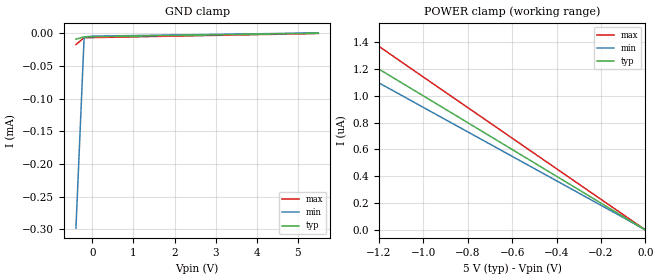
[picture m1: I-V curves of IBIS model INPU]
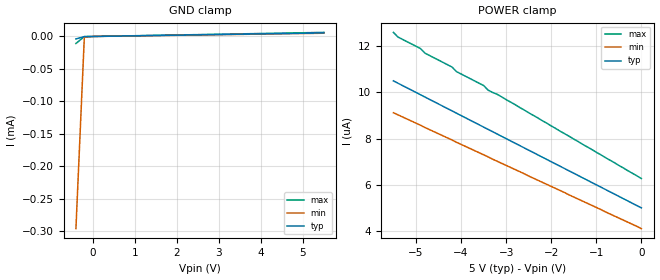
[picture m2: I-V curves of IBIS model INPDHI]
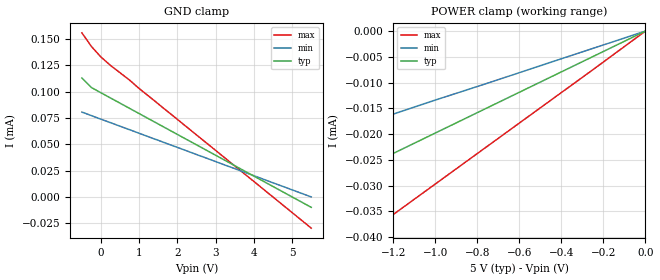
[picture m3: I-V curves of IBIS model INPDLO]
|   Texas Instruments Incorporated
|   Data Transmissions Products
|   IBIS Model for ISO723x4x
|   16DW SOIC Package
[IBIS Ver]   3.2
[Comment char]   |_char
[File name]   iso1176_5.ibs
[File Rev]   1.0
[Date]   11July08
[Source]   File originated at Texas Instruments Incorporated.
   Data Transmission Products Group.
[Notes]
[Disclaimer]
(C) Copyright Texas Instruments Incorporated 2002
   All rights reserved
  Texas Instruments Incorporated hereby grants the user of this IBIS
model a non-exclusive, nontransferable license to use this IBIS model
under the following terms.  Before using this IBIS model, the user
should read this license.  If the user does not accept these terms,
the IBIS model should be returned to Texas Instruments within 30 days.
  The user is granted this license only to use the IBIS model and
is not granted rights to sell, load, rent, lease or license the IBIS
model in whole or in part, or in modified form to anyone other than
user.  User may modify the IBIS model to suit its specific applications
but rights to derivative works and such modifications shall belong to
Texas Instruments.
  This IBIS model is provided on an "AS IS" basis and Texas Instruments
makes absolutely no warranty with respect to the information contained
herein.  TEXAS INSTRUMENTS DISCLAIMS AND CUSTOMER WAIVES ALL WARRANTIES,
EXPRESS OR IMPLIED, INCLUDING WARRANTIES OF MERCHANTABILITY OR FITNESS
FOR A PARTICULAR PURPOSE. The entire risk as to quality and performance
is with the Customer. ACCORDINGLY, IN NO EVENT SHALL THE COMPANY BE LIABLE
FOR ANY DAMAGES, WHETHER IN CONTRACT OR TORT,INCLUDING ANY LOST PROFITS
OR OTHER INCIDENTAL, CONSEQUENTIAL, EXEMPLARY, OR PUNITIVE DAMAGES ARISING
OUT OF THE USE OR APPLICATION OF THE IBIS model provided in this package.
Further, Texas Instruments reserves the right to discontinue or make changes
without notice to any product herein to improve reliability, function, or
design. Texas Instruments does not convey any license under patent rights
or any other intellectual property rights, including those of third parties.
Contact Texas Instruments at ATTN:DATA TRANSMISSIONS
[Copyright]   Copyright 2002, Texas Instruments, All Rights Reserved
[Component]   ISO1176DW
[Manufacturer]  Texas Instruments Incorporated
[Package]
|   typ   min   max
R_pkg   0.04817   0.03432   0.09530
L_pkg   2.4595nH   1.6904nH   4.7034nH
C_pkg   0.847pF   0.428pF   1.397pF
[Pin]   signal_name   model_name   R_pin   L_pin   C_pin
1   VCC1   POWER   0.03455  3.39778n  0.89677p
2   GND1   GND   0.03432  3.12613n  0.84706p
3   R   OUTR   0.04265  1.85523n  0.57831p
4   REB   INPU   0.03948  1.69049n  0.59300p
5   DE   INPDHI   0.03943  1.70546n  0.55709p
6   D   INPU   0.04257  1.86953n  0.56379p
7   PV   INPDLO   0.04783  1.99000n  0.60148p
8   GND1   GND   0.03740  4.70338n  1.39696p
9   GND2   GND   0.03763  4.61305n  1.39587p
10   ISODE   OUTDE   0.08703  5.01514n  1.58483p
11   NC   NC   0.07132  2.45946n  0.43321p
12   A   DRVR/REC_BI   0.06147  2.13194n  0.42769p
13   B   DRVR/REC_BI   0.07288  2.39260n  0.48001p
14   NC   NC   0.09530  3.03704n  0.47622p
15   GND2   GND   0.04817  4.23145n  0.93567p
16   VCC2   POWER   0.04790  4.51154n  0.99405p
[Diff_pin]   inv_pin   vdiff   tdelay_typ   tdelay_min   tdelay_max
| The 'A' pin is Diff_pin and the 'B' pin is the inv_pin
12   13   0.200   0 0 0
| Models and submodels in the file (6): INPU (Input), INPDHI (Input), INPDLO (Input), OUTDE (3-state), OUTR (3-state), DRVR/REC_BI (I/O)
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|   Driver Input / Receiver Enable Model
[Model]   INPU
Model_type   Input
|Signals   REB,D
Vinh = 2.0
Vinl = 0.8
|   typ   min   max
C_comp   1.3pF   1.1pF   1.5pF
|   typ   min   max
[Temperature Range]   27   -40   85
[Voltage range]   5.0V   4.5V   5.5V
[GND_clamp]
|   Voltage   I(typ)   I(min)   I(max)
-400mV    -8.71uA    -298uA     -16.9uA
-200mV    -5.2uA     -5.27uA    -6.5uA
0V        -5uA       -4.1uA     -6.27uA
5.5V      500nA      913nA      27.5pA
[Power_clamp]
| Note that the[POWER_clamp]voltage table is referenced to Vcc
| and is calculated using Vtable=Vcc - Vmeasured.
|   Voltage   I(typ)   I(min)   I(max)
-5.5V     5.498uA    5.021uA    6.28uA
-1.7V     1.699uA    1.552uA    1.939uA
-1.6V     1.599uA    1.461uA    1.825uA
-1.5V     1.499uA    1.369uA    1.711uA
-1.4V     1.399uA    1.278uA    1.597uA
-1.3V     1.299uA    1.187uA    1.483uA
0V        0A         0A         0A
|   Driver Enable
[Model]   INPDHI
Model_type   Input
|Signals   DE
Vinh = 2.0
Vinl = 0.8
|   typ   min   max
C_comp   1.3pF   1.1pF   1.5pF
|   typ   min   max
[Temperature Range]   27   -40   85
[Voltage range]   5.0V   4.5V   5.5V
[GND_clamp]
|   Voltage   I(typ)   I(min)   I(max)
-400mV    -3.79uA    -296uA     -10.8uA
-200mV    -202nA     -1.2uA     -230nA
0V        0A         0A         0A
5.5V      5.5uA      5.02uA     6.27uA
[Power_clamp]
| Note that the[POWER_clamp]voltage table is referenced to Vcc
| and is calculated using Vtable=Vcc - Vmeasured.
|   Voltage   I(typ)   I(min)   I(max)
-5.5V     10.5uA     9.12uA     12.6uA
-5.4V     10.4uA     9.03uA     12.4uA
-4.9V     9.9uA      8.58uA     11.9uA
-4.8V     9.8uA      8.48uA     11.7uA
-4.2V     9.2uA      7.94uA     11.1uA
-4.1V     9.1uA      7.84uA     10.9uA
-3.5V     8.5uA      7.3uA      10.3uA
-3.4V     8.4uA      7.21uA     10.1uA
-3.1V     8.1uA      6.93uA     9.81uA
0V        5uA        4.1uA      6.27uA
|   PV Enable Model
[Model]   INPDLO
Model_type   Input
|Signals   PV
Vinh = 2.0
Vinl = 0.8
|   typ   min   max
C_comp   1.3pF   1.1pF   1.5pF
|   typ   min   max
[Temperature Range]   27   -40   85
[Voltage range]   5.0V   4.5V   5.5V
[GND_clamp]
|   Voltage   I(typ)   I(min)   I(max)
-500mV    113.1uA    80.7uA     156uA
-250mV    104uA      77.3uA     143uA
0V        99.01uA    73.9uA     133uA
250mV     94.06uA    70.6uA     125uA
750mV     84.16uA    63.9uA     111uA
1V        79.21uA    60.5uA     103uA
5.5V      -9.901uA   -20.7pA    -29.7uA
[Power_clamp]
| Note that the[POWER_clamp]voltage table is referenced to Vcc
| and is calculated using Vtable=Vcc - Vmeasured.
|   Voltage   I(typ)   I(min)   I(max)
-5.5V     -108.9uA   -73.9uA    -170uA
-3V       -59.41uA   -40.3uA    -89.4uA
-2.75V    -54.45uA   -37uA      -81.9uA
-2V       -39.6uA    -26.9uA    -59.4uA
-1.75V    -34.65uA   -23.5uA    -52uA
-1.5V     -29.7uA    -20.2uA    -44.5uA
-1.25V    -24.75uA   -16.8uA    -37.1uA
0V        0A         0A         0A
